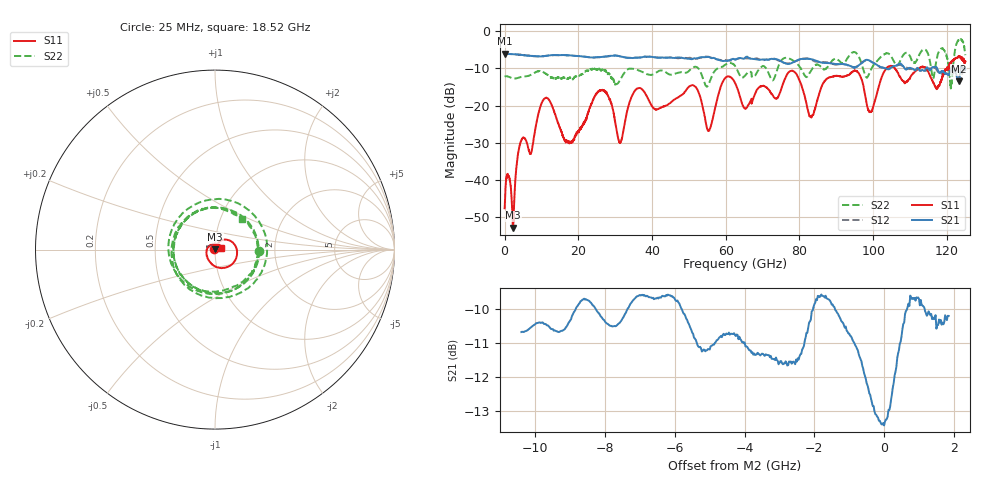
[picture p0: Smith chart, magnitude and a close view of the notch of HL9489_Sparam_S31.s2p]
! 2/28/2024 4:17:06 PM
! H:\PROTOTYPE_DATA\2-2024-110GHZ\4A-S31.S2P
! CHANNEL.1
! TR.MEASUREMENT
! CORRECTED.DATA
# GHZ S RI R 50.0
! FREQ.GHZ  S11RE  S11IM  S21RE  S21IM  S12RE  S12IM  S22RE  S22IM
!; PortSelection: Port_12
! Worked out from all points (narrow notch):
!   5000 points, 25 MHz to 125 GHz, reference 50 ohm
!   highest |S21| = -6.01 dB at 25 MHz (marker M1); lowest = -13.4 dB at 123.2 GHz (marker M2)
!   notch at M2: 6.0 dB deep, 1.73 GHz wide at half that depth
!   lowest |S11| = -52.8 dB at 2.35 GHz (marker M3), VSWR 1.00, Z = 50.2 + j0.16 ohm
!   |S11| at or under -10 dB: start of sweep to 103.5 GHz; 105.9 GHz to 112.4 GHz (6.526 GHz wide, 5.98 % of centre); 114.4 GHz to 120 GHz (5.522 GHz wide, 4.71 % of centre)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
!   |S22| runs from -15.4 to -2.1 dB; largest |S21 - S12| = 0.15
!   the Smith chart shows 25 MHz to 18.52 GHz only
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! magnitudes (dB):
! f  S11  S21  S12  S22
! 25 MHz  -47.6  -6.0  -6.0  -12.2
! 2.35 GHz  -52.8  -6.2  -6.2  -12.7
! 4.325 GHz  -30.0  -6.3  -6.3  -12.3
! 7.175 GHz  -32.8  -6.6  -6.6  -11.7
! 10.7 GHz  -18.3  -6.7  -6.7  -11.1
! 20.88 GHz  -25.8  -6.7  -6.7  -11.6
! 26.12 GHz  -15.9  -6.9  -7.0  -10.5
! 31.3 GHz  -30.0  -6.7  -6.7  -13.2
! 35.8 GHz  -15.5  -7.1  -7.1  -10.3
! 41.7 GHz  -20.9  -7.1  -7.1  -10.8
! 51.3 GHz  -14.6  -7.3  -7.5  -9.7
! 55.42 GHz  -26.7  -6.9  -6.9  -14.1
! 62.52 GHz  -13.9  -7.6  -7.5  -9.3
! 65.38 GHz  -20.8  -7.0  -7.3  -11.8
! 78.28 GHz  -10.7  -8.4  -8.3  -7.9
! 83.35 GHz  -22.9  -7.6  -7.7  -10.3
! 94.97 GHz  -10.6  -9.8  -9.7  -5.6
! 99.35 GHz  -21.8  -8.1  -8.1  -10.4
! 104.2 GHz  -9.5  -10.2  -9.9  -6.0
! 121 GHz  -8.4  -10.3  -10.5  -15.4
! 123.2 GHz  -6.7  -13.4  -11.5  -2.4
! 125 GHz  -8.1  -10.2  -10.0  -6.4
